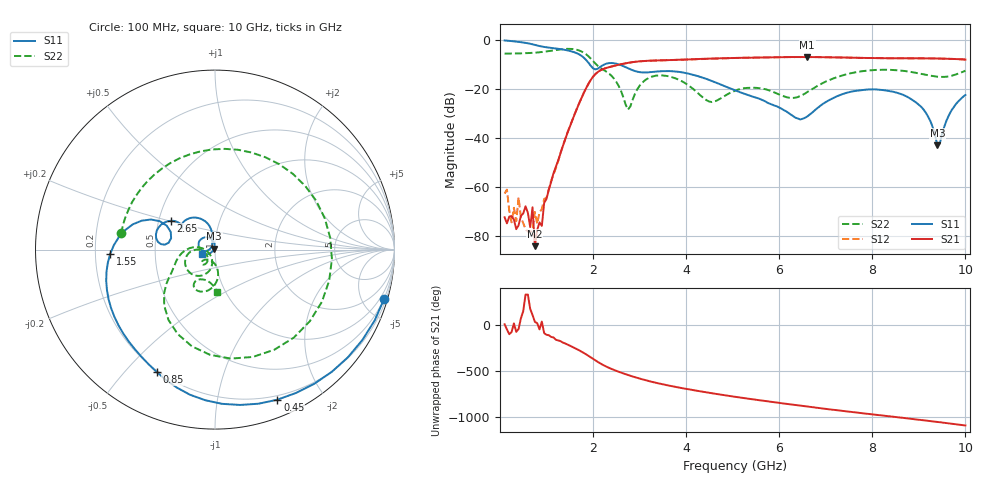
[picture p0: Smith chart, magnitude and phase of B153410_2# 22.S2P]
!  2-Port S-parameters saved by WinCal
! VAR MeasName=S-Parameters (CALIBRATED_DATA) read from VNA (N5245A)
! VAR MeasDate=2016-12-23 10:00:28
! VAR NAME=B153410_2# 22
! VAR FILENAME=B153410_2# 22.S2P
! VAR DATE=2016-12-23 10:00:28
! VAR PHYS_PORTS=1,2
# Hz S DB R 50
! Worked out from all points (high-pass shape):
!   199 points, 100 MHz to 10 GHz, reference 50 ohm
!   highest |S21| = -6.91 dB at 6.6 GHz (marker M1); lowest = -83.9 dB at 750 MHz (marker M2)
!   |S21| within 3 dB of the highest: 2.588 GHz to end of sweep
!   lowest |S11| = -42.9 dB at 9.4 GHz (marker M3), VSWR 1.01, Z = 49.5 + j0.473 ohm
!   |S11| at or under -10 dB: 1.932 GHz to 2.237 GHz (305.1 MHz wide, 14.6 % of centre); 2.564 GHz to end of sweep
!   |S22| runs from -28.3 to -3.6 dB; largest |S21 - S12| = 0.0022
!   S11 on the Smith chart (normalised r, x): 100 MHz: 0.46, -7.02; 450 MHz: 0.16, -1.49; 850 MHz: 0.19, -0.61; 1.55 GHz: 0.26, -0.02; 2.65 GHz: 0.58, +0.20; 10 GHz: 0.87, -0.05
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1e8  -0.16 -16.1  -72.18 6.7  -62.50 130.9  -5.51 170.2
2.5e8  -0.42 -39.0  -71.68 -77.4  -74.23 -154.4  -5.51 155.3
3.5e8  -0.63 -53.5  -77.02 -75.2  -73.76 -170.7  -5.47 145.1
4e8  -0.75 -60.5  -75.47 -45.4  -64.07 56.5  -5.45 139.8
4.5e8  -0.86 -67.4  -71.62 70.2  -72.11 -153.9  -5.42 134.4
6.5e8  -1.50 -93.7  -76.18 172.1  -78.41 -94.0  -5.26 111.1
7e8  -1.72 -99.8  -68.10 106.6  -77.21 114.2  -5.21 104.9
7.5e8  -1.96 -105.4  -83.94 33.4  -69.99 -63.7  -5.14 98.3
8.5e8  -2.44 -115.6  -74.28 -48.7  -70.18 -38.9  -4.98 84.4
1.3e9  -3.69 -155.1  -46.10 -175.4  -45.91 -178.6  -3.81 5.9
1.55e9  -4.67 -177.8  -32.82 123.7  -32.80 123.7  -3.63 -48.2
1.75e9  -6.39 162.9  -23.65 71.4  -23.63 71.6  -4.63 -92.7
2.65e9  -10.62 147.0  -9.65 -164.7  -9.65 -164.8  -23.24 174.4
3.4e9  -12.77 144.9  -8.30 88.2  -8.31 88.2  -14.42 -138.0
4.55e9  -16.63 105.1  -7.53 -18.8  -7.55 -18.8  -25.25 -150.1
5.05e9  -20.48 100.9  -7.28 -57.6  -7.30 -57.5  -20.63 -123.1
6.6e9  -31.16 171.2  -6.91 -162.9  -6.92 -162.9  -21.21 -87.7
6.7e9  -29.69 -179.6  -6.91 -169.3  -6.93 -169.3  -20.04 -84.3
8.35e9  -20.71 134.5  -7.41 92.4  -7.41 92.5  -12.10 -114.2
9.05e9  -27.18 99.4  -7.43 51.9  -7.45 51.8  -13.76 -121.5
9.4e9  -42.86 138.4  -7.51 30.4  -7.51 30.5  -14.92 -112.3
1e10  -22.37 -159.4  -7.92 -7.4  -7.94 -7.4  -12.48 -87.0
